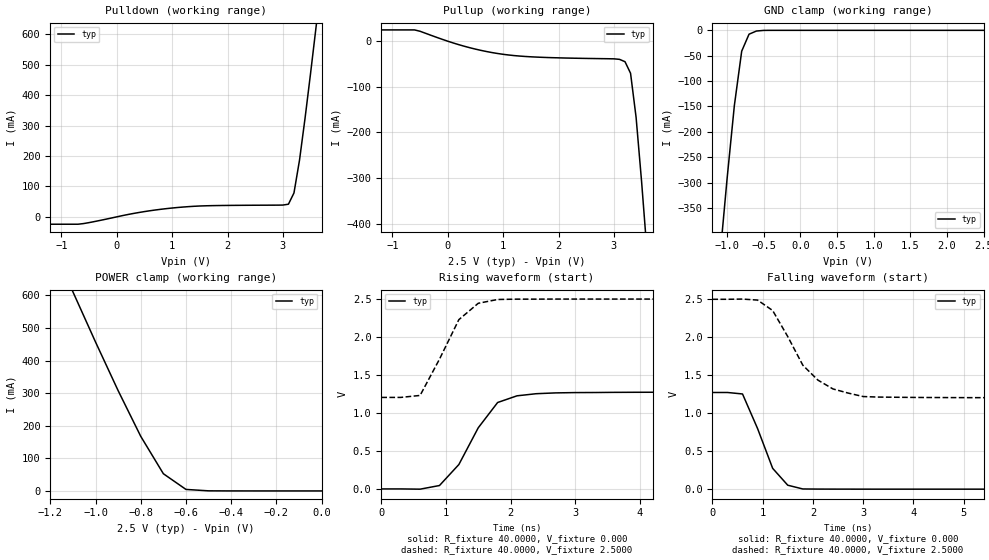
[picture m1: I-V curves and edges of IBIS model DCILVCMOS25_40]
| / 7\'7
| \ \   Xilinx Inc.
| / /
| \_\/.\   IBIS Model for Virtex-II
[IBIS ver]   2.1
[File name]   dci2540.ibs
[File Rev]   1.1
[Date]   Aug. 1, 2001
[Source]   Hspice simulations (08-01: TT, SS, FF)
[Notes]   Xilinx IBIS model for LVDCI 2.5V 40 ohms driver
[Disclaimer] The data in this model is derived from SPICE simulations using
   modeling information extracted from the target process. While
   a great deal of care has been taken to provide information
   that is accurate, this model is considered preliminary as it
   has not been verified by actual silicon measurement. Treat the
   data in this model as preliminary until actual silicon
   verification is performed.
[Copyright]   Copyright 2001, Xilinx Inc., All rights reserved
|   Component Virtex_II
[Component]   Virtex_II
[Manufacturer]   Xilinx Inc.
[Package]
| variable   typ   min   max
R_pkg   0.1000   NA   NA
L_pkg   0.8000nH   NA   NA
C_pkg   0.5000pF   NA   NA
[Pin]  signal_name   model_name   R_pin   L_pin   C_pin
io   DCILVCMOS25_40   DCILVCMOS25_40
| ins  insig   inp
| ens  ensig   inp
PGND   GND   GND
VCCO   VCCO   POWER
| Models and submodels in the file (1): DCILVCMOS25_40 (I/O)
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|   Model DCILVCMOS25_40
[Model]   DCILVCMOS25_40
Model_type   I/O
Polarity   Non-Inverting
Enable   Active-Low
Vinh = 1.7V
Vinl = 0.7V
Vmeas =   1.2000V
Cref =  35.0000pF
Rref =   1.0000M
Vref =  0.000V
C_comp   7.0000pF   NA   NA
[Temperature Range]   25.0000   NA   NA
[Voltage Range]   2.5000V   NA   NA
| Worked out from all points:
|   slope of the pulldown table from 0 to 0.375 V, typ, clamps not added: 27.8 ohm
|   slope of the pullup table from 0 to 0.375 V, typ, clamps not added: 27.7 ohm
|   GND clamp passes 1 mA (typ) near -0.57 V on its own axis
|   POWER clamp passes 1 mA (typ) near -0.52 V on its own axis
|   rising waveform, R_fixture 40.0000, V_fixture 0.000: 20-80 % time 564ps typ, NA min, NA max; typ from 0 V to 1.27 V
|   rising waveform, R_fixture 40.0000, V_fixture 2.5000: 20-80 % time 470ps typ, NA min, NA max; typ from 1.21 V to 2.5 V
|   falling waveform, R_fixture 40.0000, V_fixture 0.000: 20-80 % time 472ps typ, NA min, NA max; typ from 1.27 V to 0 V
|   falling waveform, R_fixture 40.0000, V_fixture 2.5000: 20-80 % time 760ps typ, NA min, NA max; typ from 2.5 V to 1.21 V
[Pulldown]
| voltage   I(typ)   I(min)   I(max)
-2.5V     -24.24mA   NA         NA
-700mV    -24.24mA   NA         NA
400mV     14.29mA    NA         NA
1V        29.01mA    NA         NA
1.6V      36.31mA    NA         NA
3.1V      41.57mA    NA         NA
3.2V      78.58mA    NA         NA
3.3V      186.4mA    NA         NA
3.4V      324.1mA    NA         NA
3.5V      472.2mA    NA         NA
3.6V      625.7mA    NA         NA
5V        2.888A     NA         NA
[Pullup]
| voltage   I(typ)   I(min)   I(max)
-2.5V     24.74mA    NA         NA
-600mV    24.74mA    NA         NA
300mV     -11.11mA   NA         NA
900mV     -26.96mA   NA         NA
1.6V      -34.79mA   NA         NA
3V        -38.65mA   NA         NA
3.2V      -44.91mA   NA         NA
3.3V      -70.25mA   NA         NA
3.4V      -166.8mA   NA         NA
3.5V      -308.7mA   NA         NA
3.6V      -466mA     NA         NA
5V        -2.893A    NA         NA
[GND_clamp]
| voltage   I(typ)   I(min)   I(max)
-2.5V     -2.881A    NA         NA
-1.1V     -452.1mA   NA         NA
-1V       -293.4mA   NA         NA
-900mV    -148.1mA   NA         NA
-800mV    -41.04mA   NA         NA
-700mV    -7.632mA   NA         NA
-600mV    -1.432mA   NA         NA
-500mV    -131.2uA   NA         NA
2.5V      397.5nA    NA         NA
[POWER_clamp]
| voltage   I(typ)   I(min)   I(max)
-2.5V     2.874A     NA         NA
-1.1V     610.9mA    NA         NA
-1V       456.9mA    NA         NA
-900mV    307.7mA    NA         NA
-800mV    167.5mA    NA         NA
-700mV    52.78mA    NA         NA
-600mV    4.607mA    NA         NA
-500mV    279.3uA    NA         NA
0V        397.5nA    NA         NA
[Ramp]
| variable   typ   min   max
dV/dt_r   0.7638/0.5264n   NA   NA
dV/dt_f   0.7770/0.8296n   NA   NA
R_load = 40.0000
[Rising Waveform]
R_fixture = 40.0000
V_fixture = 0.000
| time   V(typ)   V(min)   V(max)
0s        7.936uV    NA         NA
600ps     -3.2mV     NA         NA
900ps     44.76mV    NA         NA
1.2ns     321mV      NA         NA
1.5ns     805mV      NA         NA
1.8ns     1.138V     NA         NA
2.1ns     1.226V     NA         NA
2.4ns     1.254V     NA         NA
4.2ns     1.273V     NA         NA
15ns      1.273V     NA         NA
[Rising Waveform]
R_fixture = 40.0000
V_fixture = 2.5000
V_fixture_min = 2.3000
V_fixture_max = 2.7000
| time   V(typ)   V(min)   V(max)
0s        1.205V     NA         NA
300ps     1.205V     NA         NA
600ps     1.231V     NA         NA
900ps     1.708V     NA         NA
1.2ns     2.229V     NA         NA
1.5ns     2.444V     NA         NA
1.8ns     2.494V     NA         NA
2.7ns     2.5V       NA         NA
15ns      2.5V       NA         NA
[Falling Waveform]
R_fixture = 40.0000
V_fixture = 0.000
| time   V(typ)   V(min)   V(max)
0s        1.273V     NA         NA
300ps     1.273V     NA         NA
600ps     1.254V     NA         NA
900ps     797.5mV    NA         NA
1.2ns     274.1mV    NA         NA
1.5ns     52.08mV    NA         NA
1.8ns     2.714mV    NA         NA
15ns      35.61uV    NA         NA
[Falling Waveform]
R_fixture = 40.0000
V_fixture = 2.5000
V_fixture_min = 2.3000
V_fixture_max = 2.7000
| time   V(typ)   V(min)   V(max)
0s        2.5V       NA         NA
900ps     2.49V      NA         NA
1.2ns     2.352V     NA         NA
1.5ns     2.009V     NA         NA
1.8ns     1.632V     NA         NA
2.1ns     1.436V     NA         NA
2.4ns     1.319V     NA         NA
3ns       1.22V      NA         NA
5.1ns     1.205V     NA         NA
15ns      1.205V     NA         NA
